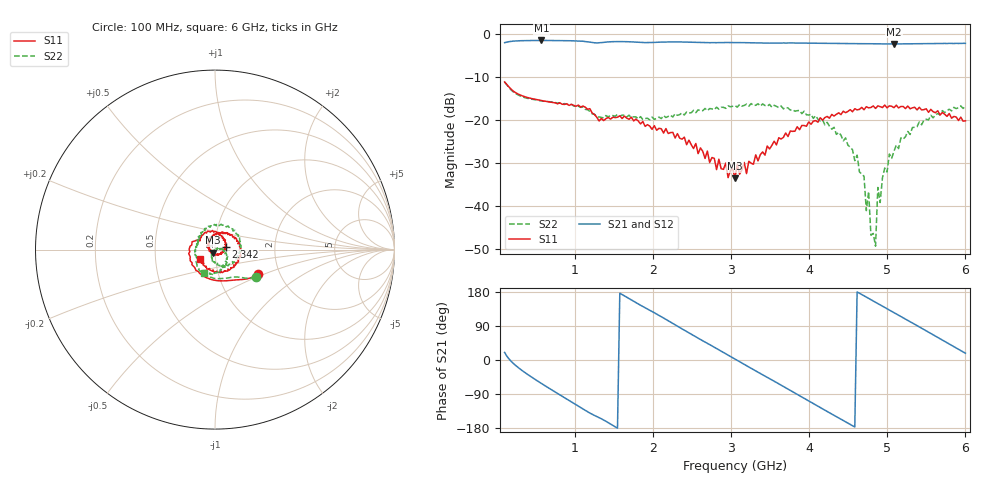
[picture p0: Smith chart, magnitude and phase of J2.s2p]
!Agilent Technologies,E8364B,MY43040379,A.07.50.67
!Agilent E8364B: A.07.50.67
!Date: Tuesday, March 24, 2026 11:04:37
!Correction: S11(Full 2 Port(1,2))
!S21(Full 2 Port(1,2))
!S12(Full 2 Port(1,2))
!S22(Full 2 Port(1,2))
!S2P File: Measurements: S11, S21, S12, S22:
# Hz S  dB  R 50
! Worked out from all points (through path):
!   201 points, 100 MHz to 6 GHz, reference 50 ohm
!   highest |S21| = -1.59 dB at 572 MHz (marker M1); lowest = -2.4 dB at 5.085 GHz (marker M2)
!   group delay of S21, straight-line fit = 328 ps
!   lowest |S11| = -33.5 dB at 3.05 GHz (marker M3), VSWR 1.04, Z = 48.8 - j1.71 ohm
!   |S11| at or under -10 dB: start of sweep to end of sweep
!   |S22| runs from -49.3 to -11.3 dB; largest |S21 - S12| = 0.0046
!   S11 on the Smith chart (normalised r, x): 100 MHz: 1.55, -0.46; 2.342 GHz: 1.12, +0.04; 6 GHz: 0.85, -0.09
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1e8  -11.22 -29.7  -2.10 20.0  -2.11 19.7  -11.27 -34.3
2.77e8  -14.05 -59.3  -1.67 -20.5  -1.69 -20.7  -14.27 -52.0
5.72e8  -15.53 -98.0  -1.59 -62.0  -1.61 -62.3  -15.63 -76.7
1.103e9  -16.81 179.6  -1.78 -129.2  -1.80 -129.4  -17.06 -135.4
1.575e9  -19.08 119.4  -1.85 176.3  -1.87 176.2  -19.16 -170.1
2.0765e9  -21.98 56.5  -1.99 117.8  -2.01 117.5  -19.37 154.5
2.342e9  -24.26 15.5  -1.93 85.8  -1.95 85.6  -18.79 137.8
3.05e9  -33.52 -123.9  -2.08 2.6  -2.09 2.3  -16.70 65.4
3.6105e9  -24.16 127.7  -2.19 -62.9  -2.21 -63.0  -17.19 1.7
4.053e9  -20.32 79.4  -2.22 -115.1  -2.24 -115.2  -19.68 -53.7
4.6135e9  -17.69 21.0  -2.33 179.6  -2.35 179.5  -28.19 -120.2
4.702e9  -17.66 14.8  -2.35 169.3  -2.36 169.2  -33.09 -147.6
4.7315e9  -16.97 13.8  -2.34 166.0  -2.36 165.9  -41.05 -142.7
4.761e9  -17.22 6.3  -2.35 162.4  -2.37 162.3  -36.65 -130.5
4.7905e9  -17.14 6.0  -2.35 159.0  -2.38 158.9  -46.77 -154.4
4.8495e9  -17.36 -0.4  -2.37 152.2  -2.38 152.0  -49.31 90.1
4.879e9  -16.76 -1.0  -2.37 148.8  -2.39 148.7  -35.69 30.3
4.9085e9  -16.94 -8.6  -2.37 145.3  -2.39 145.1  -39.19 -0.8
5.0265e9  -16.76 -15.6  -2.40 131.7  -2.41 131.6  -27.94 8.9
5.0855e9  -17.18 -22.8  -2.40 124.8  -2.42 124.8  -27.30 5.6
5.4985e9  -17.45 -72.7  -2.31 77.0  -2.33 76.8  -19.88 -57.3
6e9  -20.23 -146.2  -2.26 17.9  -2.28 17.8  -16.88 -114.7
